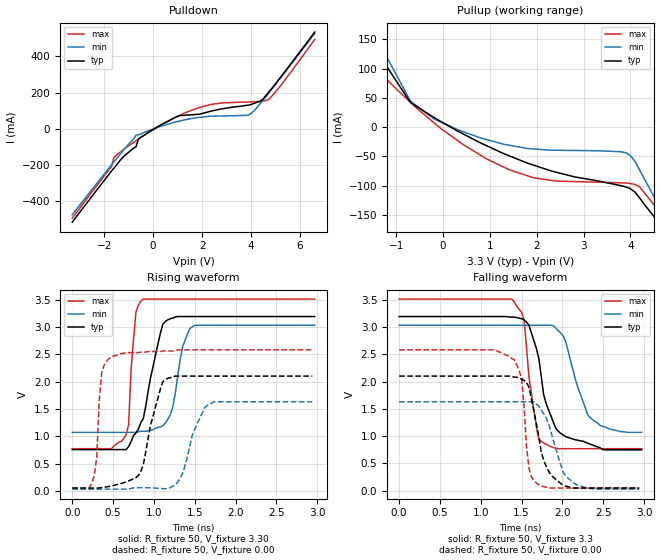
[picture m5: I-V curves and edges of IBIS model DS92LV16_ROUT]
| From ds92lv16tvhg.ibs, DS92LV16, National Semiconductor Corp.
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[Model]   DS92LV16_ROUT
Model_type Output
Polarity Non-Inverting
Vref=0.0
Vmeas=1.65
Rref=500
Cref=50p
C_comp   3.122pF   3.122pF   3.122pF
[Temperature Range] 25   85   -40
[Voltage Range]   3.3   3.15   3.45
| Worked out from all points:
|   slope of the pulldown table from 0 to 0.495 V, typ, clamps not added: 12.9 ohm
|   slope of the pullup table from 0 to 0.495 V, typ, clamps not added: 22.7 ohm
|   falling waveform, R_fixture 50, V_fixture 3.3: 20-80 % time 233ps typ, 237ps min, 126ps max; typ from 3.19 V to 0.75 V
|   rising waveform, R_fixture 50, V_fixture 3.30: 20-80 % time 214ps typ, 137ps min, 68.3ps max; typ from 0.755 V to 3.19 V
|   falling waveform, R_fixture 50, V_fixture 0.00: 20-80 % time 179ps typ, 199ps min, 82.4ps max; typ from 2.1 V to 0.05 V
|   rising waveform, R_fixture 50, V_fixture 0.00: 20-80 % time 183ps typ, 199ps min, 60.3ps max; typ from 0.05 V to 2.1 V
[Pullup]
|Vtable   I(typ)   I(min)   I(max)
-3.3V     539mA      529mA      495mA
-1.7V     187mA      200mA      202mA
-1.5V     153mA      168mA      170mA
-1.4V     137mA      151mA      159mA
-1.3V     120mA      135mA      89.1mA
-700mV    42mA       44.5mA     42.5mA
300mV     -6.33mA    -4.05mA    -22.5mA
1.4V      -48.6mA    -30.8mA    -72.3mA
3.9V      -102mA     -43.6mA    -95.3mA
4.2V      -121mA     -73.5mA    -102mA
4.8V      -200mA     -167mA     -172mA
6.6V      -516mA     -476mA     -495mA
[Pulldown]
|V(pulldown)   I(typ)   I(min)   I(max)
-3.3V     -518mA     -477mA     -496mA
-1.7V     -235mA     -201mA     -210mA
-1.6V     -219mA     -184mA     -161mA
-1.2V     -154mA     -118mA     -115mA
-700mV    -101mA     -36.2mA    -66.9mA
-600mV    -57.4mA    -33.7mA    -57.4mA
1.1V      72.9mA     42.8mA     74.9mA
2.4V      98.3mA     69mA       135mA
4V        134mA      83.9mA     148mA
4.4V      154mA      143mA      151mA
4.8V      215mA      211mA      173mA
6.6V      535mA      528mA      495mA
[Ramp]
|   typ   min   max
dV/dt_r   1.26V/.185ns   0.96V/.200ns   1.5V/.060ns
dV/dt_f   1.45V/.240ns   1.15V/.260ns   1.64V/.12ns
R_load=50
[Falling Waveform]
R_fixture=50
V_fixture=3.3
V_fixture_min=3.15
V_fixture_max=3.45
0s        3.19V      3.03V      3.51V
1.38ns    3.18V      3.03V      3.51V
1.53ns    3.13V      3.03V      3.13V
1.59ns    3.03V      3.03V      2.08V
1.71ns    2.43V      3.03V      950mV
1.77ns    1.76V      3.03V      877mV
1.95ns    1.09V      2.93V      771mV
2.04ns    991mV      2.73V      771mV
2.31ns    873mV      1.39V      771mV
2.97ns    750mV      1.07V      771mV
[Rising Waveform]
R_fixture=50
V_fixture=3.30
V_fixture_min=3.15
V_fixture_max=3.45
0s        755mV      1.07V      771mV
660ps     755mV      1.07V      1.03V
690ps     810mV      1.07V      1.21V
720ps     900mV      1.07V      2.21V
780ps     1.06V      1.07V      3.27V
870ps     1.32V      1.09V      3.51V
1.17ns    3.13V      1.31V      3.51V
1.35ns    3.19V      2.63V      3.51V
1.5ns     3.19V      3.03V      3.51V
2.97ns    3.19V      3.03V      3.51V
[Falling Waveform]
R_fixture=50
V_fixture=0.00
V_fixture_min=0.00
V_fixture_max=0.00
0s        2.1V       1.63V      2.58V
1.35ns    2.1V       1.63V      2.46V
1.5ns     2.05V      1.63V      2.06V
1.56ns    1.98V      1.63V      814mV
1.59ns    1.9V       1.63V      415mV
1.65ns    1.46V      1.63V      185mV
1.77ns    560mV      1.41V      77.9mV
1.98ns    133mV      467mV      50.7mV
2.19ns    50.4mV     102mV      50.7mV
2.94ns    50.4mV     30mV       50.7mV
[Rising Waveform]
R_fixture=50
V_fixture=0.00
V_fixture_min=0.00
V_fixture_max=0.00
0s        50.3mV     30.2mV     50.5mV
270ps     50.3mV     30.2mV     284mV
300ps     50.3mV     30.2mV     615mV
360ps     59.3mV     30.2mV     2.16V
480ps     88.6mV     30.2mV     2.45V
840ps     355mV      58mV       2.54V
1.17ns    2.06V      41.8mV     2.56V
1.35ns    2.1V       317mV      2.58V
1.65ns    2.1V       1.56V      2.58V
2.94ns    2.1V       1.63V      2.58V
